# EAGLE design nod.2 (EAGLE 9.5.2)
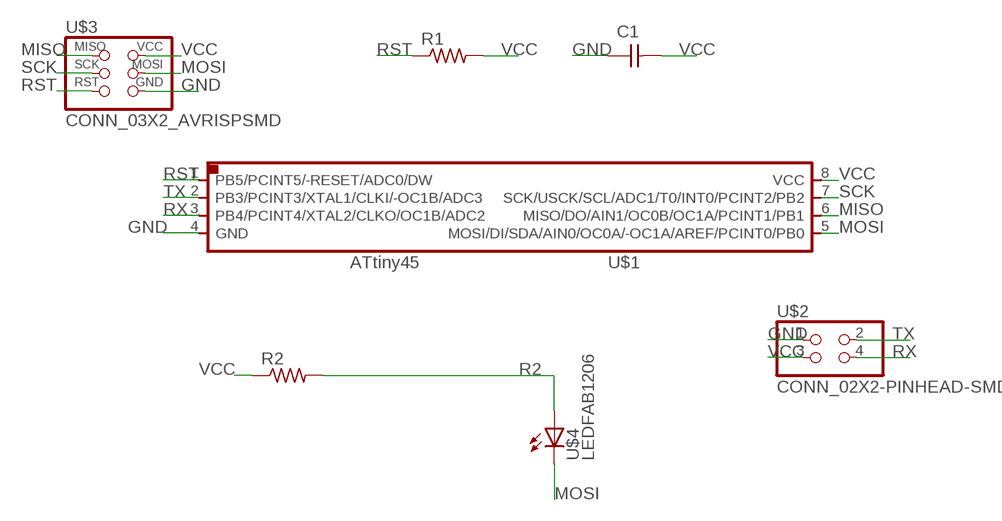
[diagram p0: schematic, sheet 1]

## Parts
C1  CAP_UNPOLARIZEDFAB  [C1206FAB]
R1  R1206FAB  [R1206FAB]
R2  R1206FAB  [R1206FAB]
U$1  UC_ATTINY45SI  [SOIC8]
U$2  CONN_02X2-PINHEAD-SMD  [2X02SMD]
U$3  CONN_03X2_AVRISPSMD  [2X03SMD]
U$4  LEDFAB1206  [LED1206FAB]

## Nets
GND: C1.1 U$1.4(GND) U$2.1 U$3.6(GND)
MISO: U$1.6(MISO/DO/AIN1/OC0B/OC1A/PCINT1/PB1) U$3.1(MISO)
MOSI: U$1.5(MOSI/DI/SDA/AIN0/OC0A/-OC1A/AREF/PCINT0/PB0) U$3.4(MOSI) U$4.2(C)
R2: R2.2 U$4.1(A)
RST: R1.1 U$1.1(PB5/PCINT5/-RESET/ADC0/DW) U$3.5(RST)
RX: U$1.3(PB4/PCINT4/XTAL2/CLKO/OC1B/ADC2) U$2.4
SCK: U$1.7(SCK/USCK/SCL/ADC1/T0/INT0/PCINT2/PB2) U$3.3(SCK)
TX: U$1.2(PB3/PCINT3/XTAL1/CLKI/-OC1B/ADC3) U$2.2
VCC: C1.2 R1.2 R2.1 U$1.8(VCC) U$2.3 U$3.2(VCC)

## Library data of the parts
C1 = eagle_fab:CAP_UNPOLARIZED
R1 R2 = eagle_fab:R: Resistor (US Symbol)
U$1 = eagle_fab:UC_ATTINY45
U$2 = eagle_fab:CONN_02X2-PINHEAD-SMD
U$3 = eagle_fab:CONN_03X2_AVRISP
U$4 = eagle_fab:LED: LED

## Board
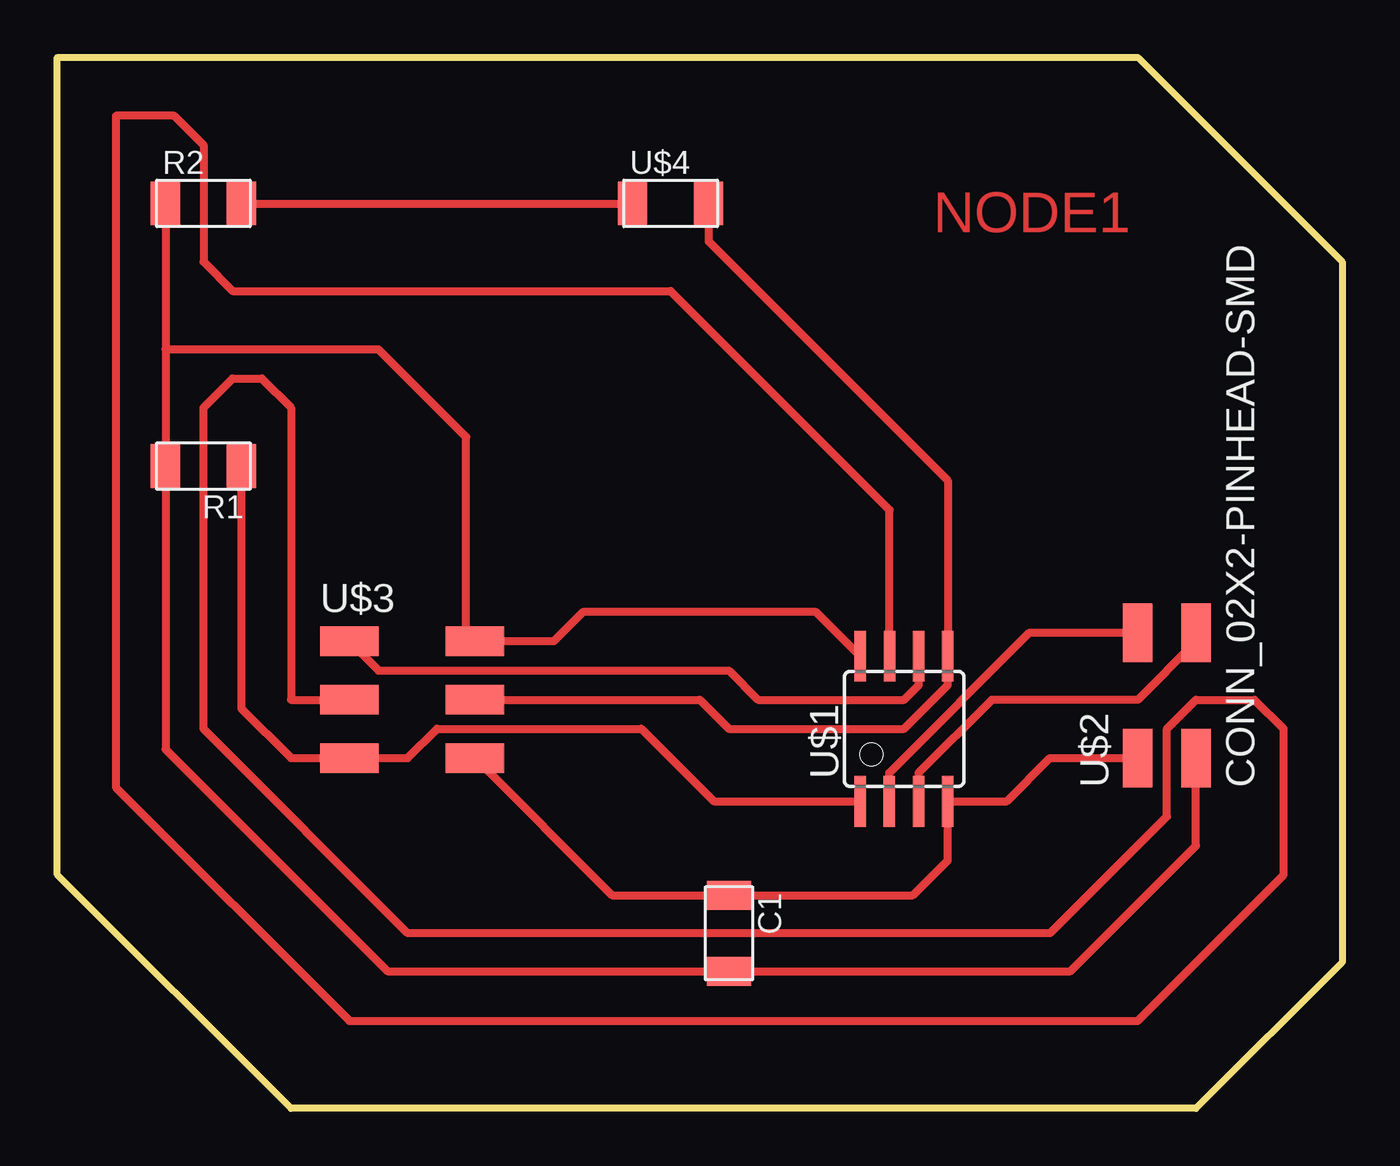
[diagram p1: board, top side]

Size 55.88 x 45.72 mm. Coordinates in mm from the lower left corner, seen from the top.
Outline: 0,45.72 46.99,45.72 55.88,36.83 55.88,6.35 49.53,0 10.16,0 0,10.16 0,45.72
Copper layers (1*16): Top 0.035mm / dielectric 1.5mm / Bottom 0.035mm
Design rules "default": minimum track width 6mil, minimum drill 0.35mm, track to track 6mil, track to pad 6mil, pad to pad 6mil, via to via 6mil, smd to smd 6mil, copper to edge 40mil, drill to drill 6mil, minimum pad ring 10mil, minimum via ring 8mil, stop-mask expansion 4mil, vias tented up to drill 0mil, thermal gap 10mil

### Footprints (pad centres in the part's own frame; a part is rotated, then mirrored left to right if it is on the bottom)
C1206FAB = smd 1.27 x 1.905: 1 -1.651,0; 2 1.651,0
R1206FAB = smd 1.27 x 1.905: 1 -1.651,0; 2 1.651,0
SOIC8 = smd 0.5 x 2.2: 1 -1.905,-3.154; 2 -0.645,-3.154; 3 0.625,-3.154; 4 1.895,-3.154; 5 1.905,3.154; 6 0.635,3.154; 7 -0.635,3.154; 8 -1.905,3.154
2X02SMD = smd 2.54 x 1.27: 1 -2.54,1.27; 2 2.92,1.27; 3 -2.54,-1.27; 4 2.92,-1.27
2X03SMD = smd 2.54 x 1.27: 1 -2.54,2.54; 2 2.92,2.54; 3 -2.54,0; 4 2.92,0; 5 -2.54,-2.54; 6 2.92,-2.54
LED1206FAB = smd 1.27 x 1.905: 1 -1.651,0; 2 1.651,0

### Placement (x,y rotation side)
C1  29.21,7.62 270 top
R1  6.35,27.94 180 top
R2  6.35,39.37 0 top
U$1  36.83,16.51 0 top
U$2  48.26,17.78 90 top
U$3  15.24,17.78 0 top
U$4  26.67,39.37 0 top

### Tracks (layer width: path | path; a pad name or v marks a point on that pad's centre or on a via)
GND
  Top 0.356: U$2.1 43.18,15.24 41.3,13.36 U$1.4 38.73,10.78 37.21,9.27 C1.1 24.13,9.27 U$3.6
MISO
  Top 0.356: U$3.1 13.97,19.05 29.21,19.05 30.48,17.78 36.83,17.78 37.47,18.41 U$1.6
MOSI
  Top 0.356: U$4.2 28.32,37.72 38.73,27.3 U$1.5 38.73,18.41 36.83,16.51 29.21,16.51 27.94,17.78 U$3.4
R2
  Top 0.356: R2.2 U$4.1
RST
  Top 0.356: U$1.1 28.55,13.36 25.4,16.51 16.51,16.51 15.24,15.24 U$3.5 10.16,15.24 8,17.4 R1.1
RX
  Top 0.356: U$2.4 49.53,20.32 46.99,17.78 40.64,17.78 37.45,14.59 U$1.3
SCK
  Top 0.356: U$1.7 36.2,26.03 26.67,35.56 7.62,35.56 6.35,36.83 6.35,41.91 5.08,43.18 2.54,43.18 2.54,13.97 12.7,3.81 46.99,3.81 53.34,10.16 53.34,16.51 52.07,17.78 49.53,17.78 48.26,16.51 48.26,12.7 43.18,7.62 15.24,7.62 6.35,16.51 6.35,30.48 7.62,31.75 8.89,31.75 10.16,30.48 10.16,17.78 U$3.3
TX
  Top 0.356: U$1.2 36.19,14.59 42.29,20.7 U$2.2
VCC
  Top 0.356: 5.08,38.99 R2.1 4.7,33.02 | U$2.3 49.53,11.43 44.07,5.97 C1.2 14.35,5.97 4.7,15.62 R1.2 4.7,33.02 | U$1.8 33,21.59 22.86,21.59 21.59,20.32 U$3.2 17.78,20.7 17.78,29.21 13.97,33.02 4.7,33.02

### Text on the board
Top: NODE1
